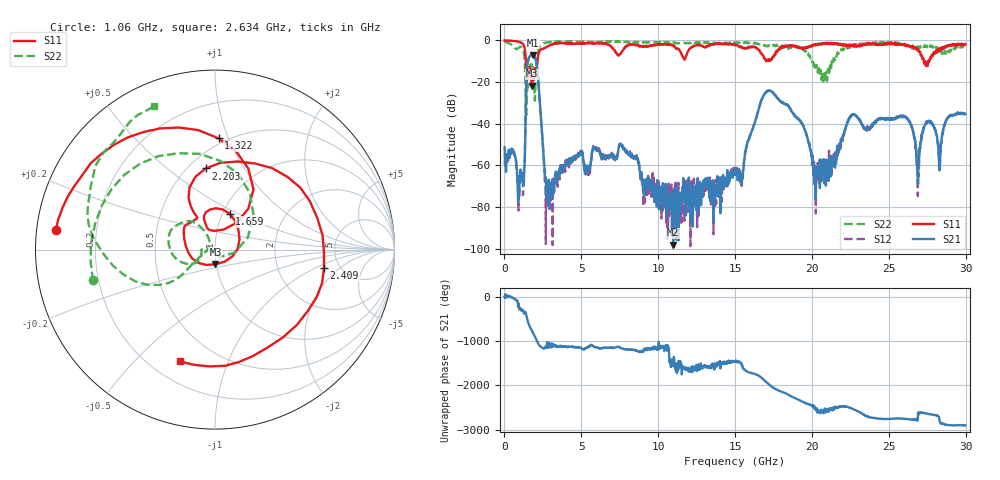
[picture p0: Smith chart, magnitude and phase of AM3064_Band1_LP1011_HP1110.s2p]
# Hz S DB R 50.0
!freq dBS11 angS11 dBS21 angS21 dBS12 angS12 dBS22 angS22
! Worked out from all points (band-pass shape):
!   1600 points, 10 MHz to 29.98 GHz, reference 50 ohm
!   highest |S21| = -6.96 dB at 1.828 GHz (marker M1); lowest = -98.1 dB at 10.98 GHz (marker M2)
!   |S21| within 3 dB of the highest: 1.533 GHz to 2.059 GHz (526.1 MHz wide, 29.3 % of centre)
!   lowest |S11| = -21.7 dB at 1.791 GHz (marker M3), VSWR 1.18, Z = 49.6 - j8.19 ohm
!   |S11| at or under -10 dB: 1.392 GHz to 2.144 GHz (751.3 MHz wide, 42.5 % of centre); 27.28285 GHz to 27.35229 GHz (69.44 MHz wide, 0.254 % of centre); 27.36 GHz to 27.57 GHz (208.9 MHz wide, 0.761 % of centre)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
!   |S22| runs from -35.9 to -0.3 dB; largest |S21 - S12| = 0.0056
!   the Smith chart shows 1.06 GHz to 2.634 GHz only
!   S11 on the Smith chart (normalised r, x): 1.06 GHz: 0.06, +0.06; 1.322 GHz: 0.46, +0.92; 1.659 GHz: 1.08, +0.45; 2.203 GHz: 0.61, +0.69; 2.409 GHz: 3.76, -1.26; 2.634 GHz: 0.32, -0.69
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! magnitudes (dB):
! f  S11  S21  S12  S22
! 10 MHz  -0.1  -51.2  -59.3  -0.3
! 1.06 GHz  -1.0  -65.8  -65.5  -3.1
! 1.322 GHz  -4.1  -57.3  -56.0  -10.8
! 1.659 GHz  -13.3  -7.5  -7.5  -12.5
! 1.791 GHz  -21.7  -7.0  -6.9  -12.0
! 1.828 GHz  -18.5  -7.0  -7.0  -12.8
! 2.203 GHz  -6.8  -19.7  -19.7  -5.5
! 2.409 GHz  -4.2  -41.2  -41.5  -1.9
! 2.634 GHz  -3.7  -67.7  -62.3  -1.2
! 5.015 GHz  -1.4  -53.4  -53.8  -0.7
! 7.62 GHz  -5.7  -50.0  -50.4  -0.7
! 10 GHz  -2.0  -75.5  -74.3  -1.0
! 10.98 GHz  -2.6  -98.1  -71.3  -1.2
! 15 GHz  -2.1  -64.6  -62.5  -1.4
! 17.18 GHz  -9.2  -24.3  -24.1  -2.7
! 19.99 GHz  -3.0  -55.2  -56.4  -9.3
! 25 GHz  -1.3  -37.7  -37.9  -1.1
! 26.25 GHz  -2.8  -37.8  -37.5  -2.4
! 26.89 GHz  -4.3  -68.7  -74.7  -3.5
! 27.49 GHz  -10.8  -39.1  -39.5  -3.0
! 28.29 GHz  -3.9  -62.4  -57.3  -4.0
! 29.98 GHz  -1.8  -35.3  -35.0  -3.1
